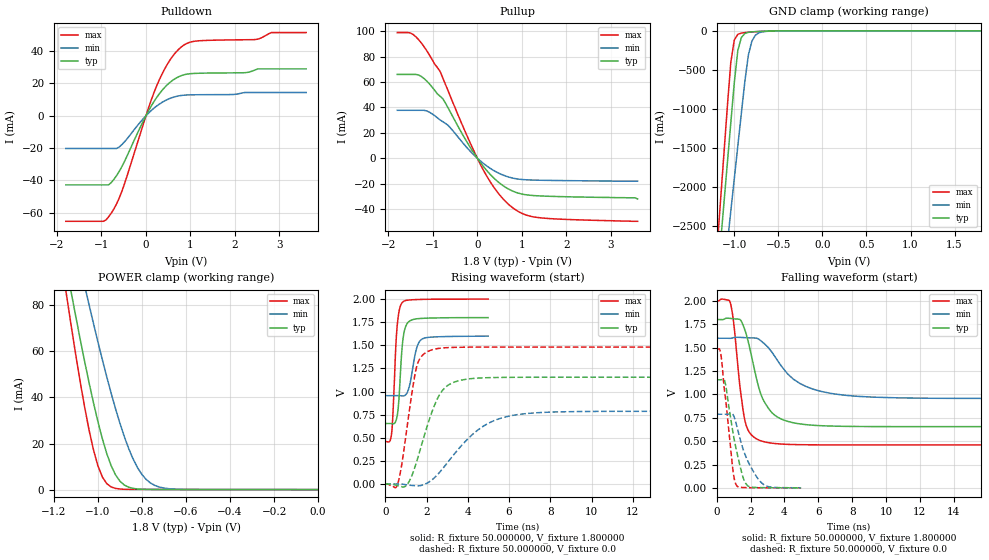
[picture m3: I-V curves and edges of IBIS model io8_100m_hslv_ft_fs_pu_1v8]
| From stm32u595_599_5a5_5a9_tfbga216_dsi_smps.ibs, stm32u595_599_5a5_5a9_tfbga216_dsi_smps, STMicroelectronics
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|   Model io8_100m_hslv_ft_fs_pu_1v8
[Model]  io8_100m_hslv_ft_fs_pu_1v8
Model_type I/O
Polarity   Non-Inverting
Enable   Active-Low
Vinl =   0.540000V
Vinh =   1.260000V
Vmeas =  0.900000V
Cref =   50.000000pF
Rref =   100.000000M
Vref =   0.0V
C_comp   3.235100pF   3.233200pF   3.282800pF
[Temperature Range]   25.000000   0.140000k   -40.000000
[Pullup Reference]   1.800000V   1.600000V   2.000000V
[Pulldown Reference]   0.0V   0.0V   0.0V
[POWER Clamp Reference]   1.800000V   1.600000V   2.000000V
[GND Clamp Reference]   0.0V   0.0V   0.0V
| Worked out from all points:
|   slope of the pulldown table from 0 to 0.27 V, typ, clamps not added: 21.7 ohm
|   slope of the pullup table from 0 to 0.27 V, typ, clamps not added: 22.6 ohm
|   GND clamp passes 1 mA (typ) near -0.51 V on its own axis
|   POWER clamp passes 1 mA (typ) near -0.86 V on its own axis
|   rising waveform, R_fixture 50.000000, V_fixture 1.800000: 20-80 % time 211ps typ, 326ps min, 197ps max; typ from 0.655 V to 1.8 V
|   rising waveform, R_fixture 50.000000, V_fixture 0.0: 20-80 % time 1.02ns typ, 2.04ns min, 582ps max; typ from 0 V to 1.16 V
|   falling waveform, R_fixture 50.000000, V_fixture 1.800000: 20-80 % time 1.09ns typ, 2.1ns min, 568ps max; typ from 1.8 V to 0.655 V
|   falling waveform, R_fixture 50.000000, V_fixture 0.0: 20-80 % time 711ps typ, 992ps min, 511ps max; typ from 1.16 V to 0 V
[Pulldown]
|Voltage   I(typ)   I(min)   I(max)
-1.8V     -42.74mA   -20.21mA   -65.25mA
-960mV    -42.74mA   -20.21mA   -65.25mA
-780mV    -41.3mA    -20.21mA   -60.25mA
-540mV    -31.39mA   -17.82mA   -46.65mA
0V        0A         0A         0A
240mV     11.28mA    6.002mA    18.38mA
480mV     19.17mA    10.02mA    31.83mA
780mV     24.67mA    12.5mA     42.21mA
1.14V     26.24mA    12.99mA    46.23mA
2.46V     28.42mA    14.38mA    47.14mA
2.82V     28.99mA    14.38mA    51.44mA
3.6V      28.99mA    14.38mA    51.44mA
[Pullup]
|Voltage   I(typ)   I(min)   I(max)
-1.8V     66.02mA    37.77mA    98.94mA
-1.44V    66.02mA    37.77mA    97.34mA
-1.14V    60.88mA    37.29mA    84.8mA
-840mV    48.91mA    30.23mA    68.54mA
-660mV    39.82mA    25.94mA    53.25mA
-300mV    16.72mA    11mA       23.08mA
120mV     -5.748mA   -3.603mA   -8.316mA
420mV     -17.18mA   -10.64mA   -25.23mA
780mV     -25.61mA   -15.48mA   -38.6mA
1.08V     -28.66mA   -16.9mA    -44.47mA
1.38V     -29.58mA   -17.26mA   -46.72mA
3.6V      -32mA      -18mA      -49.6mA
[GND_clamp]
|Voltage   I(typ)   I(min)   I(max)
-1.8V     -9.707A    -9.942A    -9.774A
-1.2V     -3.309A    -4.006A    -2.864A
-1.16V    -2.777A    -3.584A    -2.239A
-1.12V    -2.246A    -3.162A    -1.614A
-1.04V    -1.186A    -2.319A    -408.6mA
-1V       -663.9mA   -1.898A    -117.8mA
-960mV    -254mA     -1.478A    -45.14mA
-920mV    -86.03mA   -1.06A     -28.58mA
-840mV    -19.12mA   -308.9mA   -18.74mA
-800mV    -13.39mA   -130.8mA   -15.31mA
-720mV    -7.948mA   -25.37mA   -9.381mA
1.8V      0A         14.95nA    0A
[POWER_clamp]
|Voltage   I(typ)   I(min)   I(max)
-1.8V     470.9mA    433.7mA    554.6mA
-1.14V    95.28mA    122.7mA    82.88mA
-1.12V    85mA       114mA      70.34mA
-1.06V    55.55mA    88.43mA    35.73mA
-1.04V    46.38mA    80.17mA    25.83mA
-1V       29.54mA    64.14mA    10.37mA
-940mV    10.43mA    41.88mA    1.177mA
-900mV    3.66mA     28.79mA    250.5uA
-840mV    527.2uA    13.26mA    94.87uA
-800mV    153.8uA    6.55mA     88.76uA
-740mV    60.08uA    1.741mA    70.81uA
0V        0A         18.15nA    0A
[Ramp]
| variable   typ   min   max
dV/dt_r  0.69287/1.02351n   0.47201/2.03285n   0.88855/0.58126n
dV/dt_f  0.68714/1.08453n   0.38634/2.09421n   0.92439/0.56622n
R_load = 50.000000
[Rising Waveform]
R_fixture= 50.000000
V_fixture= 1.800000
V_fixture_min= 1.600000
V_fixture_max= 2.000000
|time   V(typ)   V(min)   V(max)
0s        654.9mV    956.1mV    459.5mV
310.3ps   654mV      956.3mV    551.1mV
370.4ps   652mV      956.5mV    748.8mV
550.6ps   708.7mV    956.7mV    1.633V
650.7ps   881.1mV    956.6mV    1.843V
810.8ps   1.46V      953.9mV    1.959V
1.061ns   1.736V     988.3mV    1.988V
1.512ns   1.787V     1.462V     1.995V
1.782ns   1.792V     1.568V     1.997V
4.985ns   1.8V       1.6V       2V
[Rising Waveform]
R_fixture= 50.000000
V_fixture= 0.0
V_fixture_min= 0.0
V_fixture_max= 0.0
|time   V(typ)   V(min)   V(max)
0s        492.3uV    663.5uV    443.7uV
600.6ps   -16.33mV   634uV      1.39mV
1.041ns   -8.857mV   -8.361mV   589.5mV
1.522ns   241.9mV    -18.32mV   1.27V
2.242ns   766.6mV    42.17mV    1.45V
2.683ns   984.4mV    140.5mV    1.47V
3.203ns   1.089V     285mV      1.477V
4.685ns   1.148V     616mV      1.481V
6.206ns   1.155V     744.1mV    1.481V
19.94ns   1.156V     787.5mV    1.481V
[Falling Waveform]
R_fixture= 50.000000
V_fixture= 1.800000
V_fixture_min= 1.600000
V_fixture_max= 2.000000
|time   V(typ)   V(min)   V(max)
0s        1.8V       1.6V       2V
800.8ps   1.812V     1.599V     1.984V
1.001ns   1.808V     1.607V     1.771V
1.361ns   1.802V     1.609V     1.105V
1.642ns   1.701V     1.607V     743mV
2.482ns   1.076V     1.59V      512.5mV
3.684ns   748mV      1.339V     470.4mV
4.925ns   684mV      1.116V     461.9mV
6.647ns   661.9mV    1.014V     459.8mV
19.94ns   654.9mV    956.1mV    459.5mV
[Falling Waveform]
R_fixture= 50.000000
V_fixture= 0.0
V_fixture_min= 0.0
V_fixture_max= 0.0
|time   V(typ)   V(min)   V(max)
0s        1.156V     787.5mV    1.481V
150.2ps   1.156V     787.5mV    1.487V
240.2ps   1.156V     787.6mV    1.434V
480.5ps   1.14V      787.7mV    1.012V
971ps     583.8mV    781.8mV    176.8mV
1.171ns   399.3mV    673.5mV    26.59mV
1.512ns   141.3mV    442.7mV    4.788mV
1.712ns   48.56mV    339.7mV    3.451mV
2.663ns   2.957mV    52.2mV     1.247mV
4.985ns   492.3uV    663.5uV    443.7uV
